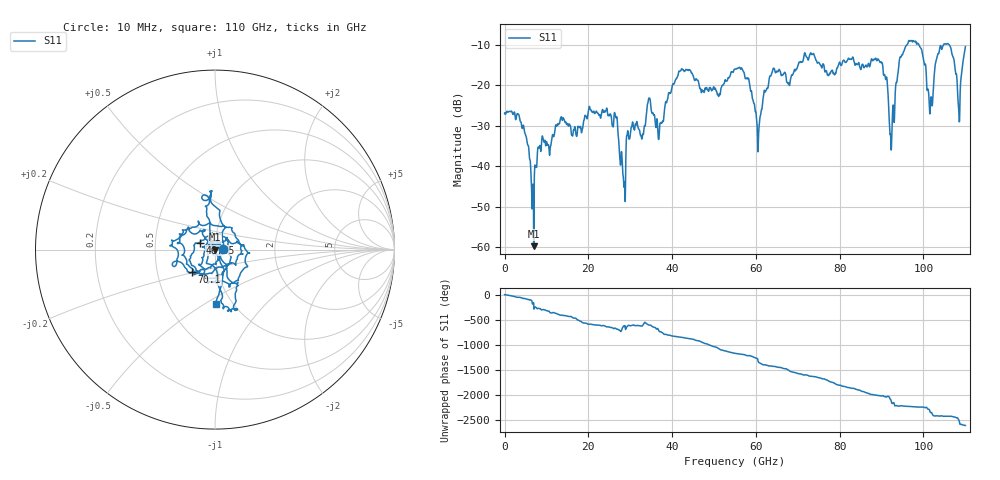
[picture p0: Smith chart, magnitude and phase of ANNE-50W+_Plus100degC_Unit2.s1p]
!Mini-Circuits Laboratory
!S-Parameters
!S1P File: Measurement
!Model: ANNE-50W+
!No.: Unit#2 (U2_100°C)
!Run / Lot / Date Code: QN2409253 /  / 2409
!Fixture: N/A
!Network Analyzer: PNA-X N5242B;  Serial number: 74314
!Pin Outs: PORT<1> = pin<1>
!TEST CONDITIONS: Z:50 OHM SYSTEM, INPUT POWER = 0dBm, TEMP:25°C
!F-F adapter to 1FT F-M cable on Port 2 head. 1mm 1 PORT SmartCal
!Date: 9/5/2024 at 12:58:36 PM
# Hz  S  dB  R  50
!Frequency  S11 dB  S11 Deg
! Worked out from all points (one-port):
!   2208 points, 10 MHz to 110 GHz, reference 50 ohm
!   lowest |S11| = -59.7 dB at 6.95 GHz (marker M1), VSWR 1.00, Z = 49.9 - j0.0211 ohm
!   |S11| at or under -10 dB: start of sweep to 96.03 GHz; 98.91 GHz to 104.8 GHz (5.851 GHz wide, 5.75 % of centre); 106.2 GHz to end of sweep
!   S11 on the Smith chart (normalised r, x): 10 MHz: 1.09, +0.00; 46.55 GHz: 0.84, +0.07; 70.1 GHz: 0.75, -0.20; 110 GHz: 0.84, -0.56
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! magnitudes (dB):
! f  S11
! 10 MHz  -26.9
! 3.5 GHz  -27.6
! 6.95 GHz  -59.7
! 8.5 GHz  -35.0
! 13.8 GHz  -28.6
! 24 GHz  -26.5
! 27.55 GHz  -38.3
! 28.45 GHz  -44.5
! 29.6 GHz  -32.6
! 34.45 GHz  -23.1
! 37.1 GHz  -29.4
! 41.3 GHz  -17.8
! 46.55 GHz  -20.5
! 55.05 GHz  -16.0
! 60.6 GHz  -33.0
! 63.85 GHz  -16.8
! 68.8 GHz  -17.3
! 70.1 GHz  -14.9
! 82.55 GHz  -13.5
! 89.7 GHz  -14.4
! 92.45 GHz  -31.5
! 94.3 GHz  -13.5
! 96.3 GHz  -9.6
! 99.25 GHz  -10.6
! 101.8 GHz  -23.1
! 104.3 GHz  -11.1
! 108.5 GHz  -26.3
! 110 GHz  -10.4
